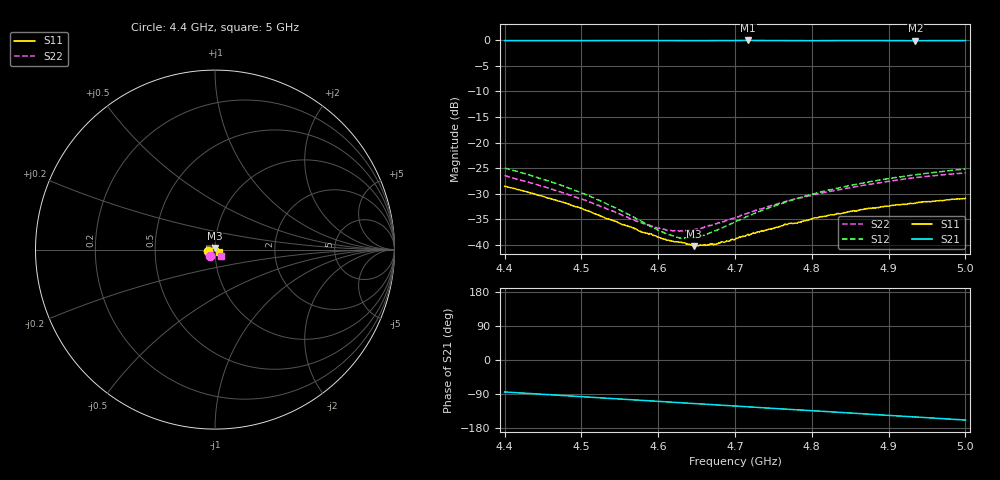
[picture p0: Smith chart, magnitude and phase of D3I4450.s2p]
! 11/4/2020 1:30:28 PM
! C:\USERS\DITOM\DESKTOP\SINGLE JUNCTION ISOLATOR DATA\4.4-5.0 GHZ (D3I4450).S2P
! CHANNEL.1
! TR.MEASUREMENT
! CORRECTED.DATA
# GHZ S RI R 50.0
! FREQ.GHZ  S11RE  S11IM  S21RE  S21IM  S12RE  S12IM  S22RE  S22IM
!; PortSelection: Port_12
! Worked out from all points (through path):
!   601 points, 4.4 GHz to 5 GHz, reference 50 ohm
!   highest |S21| = -0.09 dB at 4.717 GHz (marker M1); lowest = -0.1 dB at 4.935 GHz (marker M2)
!   lowest |S11| = -40.2 dB at 4.647 GHz (marker M3), VSWR 1.02, Z = 49.9 + j0.971 ohm
!   |S11| at or under -10 dB: start of sweep to end of sweep
!   |S22| runs from -37.3 to -25.9 dB; largest |S21 - S12| = 1
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4.4  -0.0363 -0.00876  0.0959 -0.9814  -0.045 0.0338  -0.0298 -0.0373
4.46  -0.0283 -0.00136  -0.0314 -0.9859  -0.0261 0.0322  -0.0216 -0.0281
4.5  -0.0227 0.00297  -0.1162 -0.9793  -0.015 0.0284  -0.016 -0.023
4.547  -0.0153 0.00691  -0.2145 -0.9636  -0.00403 0.0222  -0.00894 -0.0184
4.578  -0.0105 0.00827  -0.2798 -0.9478  0.00202 0.017  -0.00426 -0.016
4.592  -0.00869 0.00916  -0.3087 -0.9387  0.00435 0.0143  -0.00204 -0.0152
4.6  -0.0075 0.00927  -0.3249 -0.9329  0.0055 0.0128  -0.000886 -0.0146
4.613  -0.00557 0.00971  -0.3512 -0.9222  0.00749 0.0103  0.000961 -0.0139
4.627  -0.00356 0.0101  -0.3786 -0.9107  0.00915 0.0074  0.00321 -0.0134
4.647  -0.000659 0.00973  -0.4164 -0.8936  0.0114 0.00341  0.00599 -0.0129
4.66  0.00125 0.00997  -0.4397 -0.8824  0.0124 0.000647  0.00787 -0.0127
4.675  0.00335 0.00961  -0.4676 -0.868  0.0136 -0.00254  0.01 -0.0126
4.7  0.00666 0.0092  -0.5149 -0.8434  0.0148 -0.00805  0.0134 -0.0129
4.717  0.009 0.00905  -0.5466 -0.8249  0.0152 -0.0118  0.0157 -0.0131
4.756  0.0131 0.00711  -0.6142 -0.7727  0.0148 -0.0198  0.0207 -0.0145
4.767  0.0145 0.00649  -0.6321 -0.7577  0.0145 -0.0222  0.0222 -0.0148
4.783  0.0157 0.00567  -0.6558 -0.7358  0.0138 -0.0253  0.0241 -0.0157
4.8  0.0176 0.00436  -0.6808 -0.7112  0.0126 -0.0285  0.0257 -0.0166
4.85  0.0213 3.93e-05  -0.7543 -0.6372  0.0078 -0.0374  0.03 -0.0204
4.9  0.0235 -0.00466  -0.8191 -0.5496  0.00124 -0.0445  0.0333 -0.0252
4.935  0.0241 -0.00835  -0.8556 -0.4858  -0.00443 -0.0483  0.0351 -0.0291
5  0.0238 -0.0157  -0.9163 -0.3615  -0.0158 -0.0528  0.0356 -0.0361
